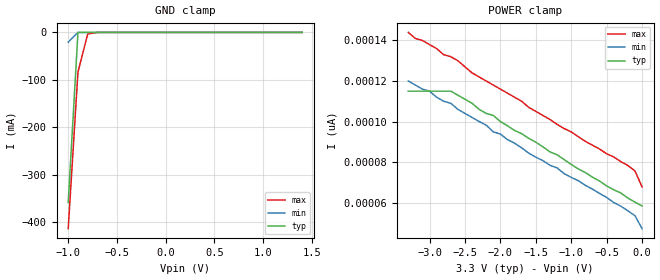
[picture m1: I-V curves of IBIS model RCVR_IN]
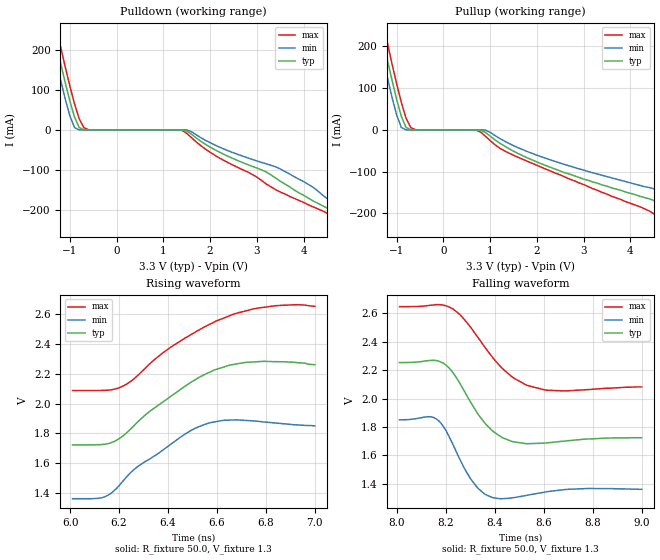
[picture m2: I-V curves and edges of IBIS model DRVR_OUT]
|   Texas Instruments Incorporated
|   Data Transmissions Products
|   IBIS Model for SN65LVDS101
|   8D SOIC Package
[IBIS Ver]   3.2
[Comment char]   |_char
[File name]   lvds101a.ibs
[File Rev]   1.1
[Date]   14Feb03
[Source]   File originated at Texas Instruments Incorporated.
   Data Transmission Products Group.
[Notes]   File was updated to include C_comp, mins and maxs
[Disclaimer]
(C) Copyright Texas Instruments Incorporated 2002
   All rights reserved
  Texas Instruments Incorporated hereby grants 1the user of this IBIS
model a non-exclusive, nontransferable license to use this IBIS model
under the following terms.  Before using this IBIS model, the user
should read this license.  If the user does not accept these terms,
the IBIS model should be returned to Texas Instruments within 30 days.
  The user is granted this license only to use the IBIS model and
is not granted rights to sell, load, rent, lease or license the IBIS
model in whole or in part, or in modified form to anyone other than
user.  User may modify the IBIS model to suit its specific applications
but rights to derivative works and such modifications shall belong to
Texas Instruments.
  This IBIS model is provided on an "AS IS" basis and Texas Instruments
makes absolutely no warranty with respect to the information contained
herein.  TEXAS INSTRUMENTS DISCLAIMS AND CUSTOMER WAIVES ALL WARRANTIES,
EXPRESS OR IMPLIED, INCLUDING WARRANTIES OF MERCHANTABILITY OR FITNESS
FOR A PARTICULAR PURPOSE. The entire risk as to quality and performance
is with the Customer. ACCORDINGLY, IN NO EVENT SHALL THE COMPANY BE LIABLE
FOR ANY DAMAGES, WHETHER IN CONTRACT OR TORT,INCLUDING ANY LOST PROFITS
OR OTHER INCIDENTAL, CONSEQUENTIAL, EXEMPLARY, OR PUNITIVE DAMAGES ARISING
OUT OF THE USE OR APPLICATION OF THE IBIS model provided in this package.
Further, Texas Instruments reserves the right to discontinue or make changes
without notice to any product herein to improve reliability, function, or
design. Texas Instruments does not convey any license under patent rights
or any other intellectual property rights, including those of third parties.
Contact Texas Instruments at ATTN:DATA TRANSMISSIONS
[Copyright]   Copyright 2002, Texas Instruments, All Rights Reserved
[Component]   LVDS101D
[Manufacturer]  Texas Instruments Incorporated
[Package]
|   typ   min   max
R_pkg   0.036   0.033   0.039
L_pkg   3.340nH   2.445nH   4.233nH
C_pkg   0.470pF   0.308pF   0.631pF
[Pin]   signal_name   model_name   R_pin   L_pin   C_pin
1   NC   NC   0.034   4.233n   0.630p
2   A   RCVR_IN   0.038   2.445n   0.309p
3   B   RCVR_IN   0.039   2.448n   0.309p
4   VBB   POWER   0.033   4.231n   0.631p
5   GND   GND   0.033   4.230n   0.630p
6   Z   DRVR_OUT   0.039   2.450n   0.308p
7   Y   DRVR_OUT   0.039   2.448n   0.309p
8   VCC   POWER   0.033   4.231n   0.630p
[Diff_pin]   inv_pin   vdiff   tdelay_typ   tdelay_min   tdelay_max
| The 'A/Y' pin is Diff_pin and the 'B/Z' pin is the inv_pin
2   3   0.050   0 0 0
7   6   NA   0 0 0
| Models and submodels in the file (2): RCVR_IN (Input), DRVR_OUT (Output_ECL)
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|   Receiver Input Model
[Model]   RCVR_IN
Model_type   Input
|Signals   A,B
Vinh = 1.4
Vinl = 1.0
|   typ   min   max
C_comp   1.8pF   1.6pF   2.0pF
|   typ   min   max
[Temperature Range]   25.0   -40   85
[Voltage range]   3.3V   3.0V   3.6V
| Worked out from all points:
|   GND clamp passes 1 mA (typ) near -0.90 V on its own axis
[GND_clamp]
|   Voltage   I(typ)   I(min)   I(max)
-1V       -359mA     -20.6mA    -414mA
-900mV    -142uA     -142uA     -83.8mA
-800mV    -980nA     -980nA     -3.28mA
-700mV    -6.76nA    -6.76nA    -128uA
1.4V      15.7pA     15.5pA     24.7pA
[Power_clamp]
| Note that the[POWER_clamp]voltage table is referenced to Vcc
| and is calculated using Vtable=Vcc - Vmeasured.
|Voltage   I(typ)   I(min)   I(max)
-3.3V     115pA      120pA      144pA
-3.2V     115pA      118pA      141pA
-3.1V     115pA      116pA      140pA
-2.8V     115pA      110pA      133pA
-2.7V     115pA      109pA      132pA
-2.4V     109pA      102pA      124pA
-2.3V     106pA      100pA      122pA
-2.1V     103pA      94.9pA     118pA
-1.8V     95.6pA     89.3pA     112pA
-200mV    62.2pA     55.9pA     78.3pA
-100mV    60.2pA     53.5pA     75.6pA
0V        58.3pA     47.1pA     67.7pA
|   Driver Output Model
[Model]   DRVR_OUT
Model_type   Output_ECL
| Signals   Y,Z
Vmeas = 2.0V   |Reference voltage for timing measurements
Cref = 1pF   |Timing specification test load capacitance value
Rref = 50
|Note: 50 Ohm load; single ended configuration
| variable   typ   min   max
C_comp   2.0pF   1.8pF   2.2pF
|   typ   min   max
[Temperature Range]   25.0   -40.0   85.0
[Voltage range]   3.3V   3.0V   3.6V
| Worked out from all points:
|   rising waveform, R_fixture 50.0, V_fixture 1.3: 20-80 % time 257ps typ, 228ps min, 296ps max; typ from 1.72 V to 2.26 V
|   falling waveform, R_fixture 50.0, V_fixture 1.3: 20-80 % time 116ps typ, 85.4ps min, 156ps max; typ from 2.25 V to 1.72 V
[Pulldown]
|Voltage I(typ)   I(min)   I(max)
-3.3V     1.467A     1.399A     1.536A
-1.5V     328mA      283mA      373mA
-1.4V     273mA      229mA      317mA
-1.3V     220mA      177mA      262mA
-1V       72.5mA     35.3mA     110mA
-800mV    5.95mA     84.1uA     28mA
-600mV    4.98uA     4.16nA     327uA
1.5V      -2.59mA    -227uA     -8.54mA
3.5V      -128mA     -97.4mA    -155mA
5.3V      -252mA     -229mA     -254mA
5.8V      -280mA     -258mA     -281mA
6.6V      -323mA     -303mA     -324mA
[Pullup]
|Voltage   I(typ)   I(min)   I(max)
| Note that the[Pullup]voltage table is referenced to Vcc
| and is calculated using Vtable=Vcc - Vmeasured.
-3.3V     1.467A     1.399A     1.536A
-1.4V     273mA      229mA      317mA
-1.3V     220mA      177mA      262mA
-1V       72.5mA     35.3mA     110mA
-800mV    5.95mA     84.1uA     28mA
-600mV    4.98uA     4.16nA     327uA
900mV     -6.21mA    -601uA     -15.5mA
2V        -77mA      -60.7mA    -85mA
4.5V      -169mA     -141mA     -201mA
5.3V      -231mA     -190mA     -247mA
6.1V      -286mA     -243mA     -291mA
6.6V      -315mA     -273mA     -318mA
[Ramp]
|   typ   min   max
dV/dt_r   0.319/263ps   0.296/227ps   0.337/305ps
dV/dt_f   0.319/115ps   0.296/85ps   0.337/155ps
R_load = 50ohm  |Note: The measurement is with 50ohm to Vtt.
[Rising Waveform]
R_fixture = 50.0
V_fixture = 1.3
V_fixture_min = 1.0
V_fixture_max = 1.6
C_fixture = 0p
L_fixture = 0n
|   V(typ)  V(min)  V(max)
6.01ns    1.724V     1.364V     2.087V
6.13ns    1.726V     1.37V      2.088V
6.17ns    1.74V      1.403V     2.092V
6.21ns    1.776V     1.47V      2.112V
6.27ns    1.867V     1.571V     2.178V
6.45ns    2.093V     1.774V     2.417V
6.57ns    2.209V     1.871V     2.529V
6.65ns    2.256V     1.889V     2.586V
6.77ns    2.28V      1.881V     2.639V
7ns       2.26V      1.851V     2.65V
[Falling Waveform]
R_fixture = 50.0
V_fixture = 1.3
V_fixture_min = 1.0
V_fixture_max = 1.6
C_fixture = 0p
L_fixture = 0n
|   V(typ)  V(min)  V(max)
8.01ns    2.254V     1.85V      2.648V
8.13ns    2.268V     1.872V     2.656V
8.17ns    2.264V     1.844V     2.662V
8.23ns    2.18V      1.672V     2.63V
8.3ns     1.977V     1.436V     2.505V
8.35ns    1.848V     1.339V     2.384V
8.39ns    1.772V     1.302V     2.292V
8.48ns    1.694V     1.302V     2.142V
8.61ns    1.687V     1.342V     2.059V
9ns       1.724V     1.36V      2.082V
